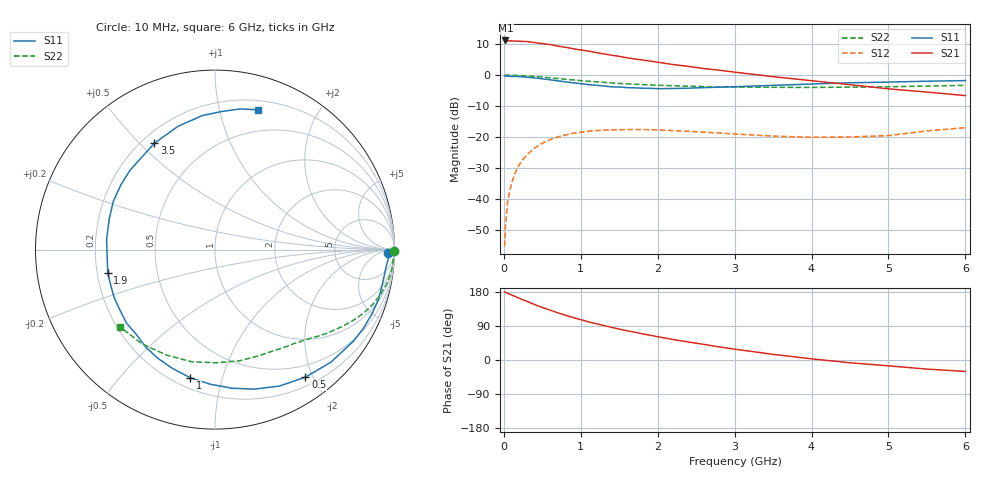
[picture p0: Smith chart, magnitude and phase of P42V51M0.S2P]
! SIEMENS Small Signal Semiconductors
! BFP182
! Si NPN RF Bipolar Junction Transistor in SOT143
! VCE = 2.5 V  IC = 1 mA
! Common Emitter S-Parameters:  March  1996
# GHz  S  MA  R  50
!  f  S11  S21  S12  S22
! GHz  MAG  ANG  MAG  ANG  MAG  ANG  MAG  ANG
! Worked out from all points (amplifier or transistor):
!   36 points, 10 MHz to 6 GHz, reference 50 ohm
!   highest |S21| = 11.2 dB at 20 MHz (marker M1)
!   |S21| within 3 dB of that: start of sweep to 978.1 MHz
!   unconditionally stable (mu >= 1): 2.633 GHz to end of sweep
!   at 250 MHz: K = 0.09, MSG = 19.1 dB, |S12| = -27.3 dB
!   at 1.4 GHz: K = 0.54, MSG = 12.1 dB, |S12| = -17.7 dB
!   at 6 GHz: K = 1.06, MAG = 3.7 dB, |S12| = -17.0 dB
!   S11 on the Smith chart (normalised r, x): 10 MHz: 40, -22; 500 MHz: 0.32, -1.89; 1 GHz: 0.26, -0.79; 1.9 GHz: 0.24, -0.10; 3.5 GHz: 0.25, +0.55; 6 GHz: 0.28, +1.31
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0.01  0.962 -1.2  3.588 179.5  0.0017 79.2  0.9987 -0.4
0.02  0.9692 -2.4  3.638 179.0  0.0035 87.0  0.9999 -0.9
0.05  0.9584 -5.7  3.599 175.8  0.0092 87.3  0.9978 -2.0
0.1  0.9526 -11.2  3.577 171.6  0.0177 82.1  0.9925 -4.2
0.15  0.9528 -17.0  3.55 167.3  0.0267 79.0  0.9914 -6.3
0.25  0.9358 -28.1  3.519 158.6  0.0432 72.9  0.9785 -10.4
0.3  0.9246 -33.5  3.489 155.0  0.0513 69.1  0.969 -12.4
0.4  0.9006 -44.1  3.361 146.4  0.066 62.9  0.9507 -16.0
0.5  0.871 -54.7  3.232 138.5  0.079 56.6  0.9282 -19.5
0.6  0.8407 -64.7  3.124 131.5  0.0902 50.8  0.904 -22.6
0.8  0.7775 -83.2  2.824 118.2  0.1074 40.8  0.856 -28.1
1  0.7271 -101.0  2.548 106.4  0.1187 32.3  0.8145 -32.6
1.1  0.7028 -109.8  2.446 100.7  0.1233 28.6  0.7958 -34.7
1.3  0.6661 -125.5  2.202 91.0  0.1284 21.6  0.7623 -38.5
1.5  0.6411 -140.3  2.013 81.6  0.1303 16.2  0.7333 -41.9
1.9  0.6112 -167.8  1.688 65.4  0.1304 7.4  0.6942 -48.3
2.2  0.6067 174.7  1.482 54.1  0.1263 2.9  0.6734 -53.0
2.8  0.6373 145.0  1.199 34.5  0.1156 -2.6  0.6445 -63.3
3.5  0.682 119.7  0.943 14.9  0.103 -2.8  0.6345 -77.6
4.5  0.7505 95.3  0.699 -7.3  0.0996 6.7  0.6382 -101.9
5.5  0.7962 79.8  0.531 -24.0  0.125 15.9  0.6646 -128.1
6  0.8146 73.0  0.466 -30.2  0.1408 14.7  0.6823 -140.9
